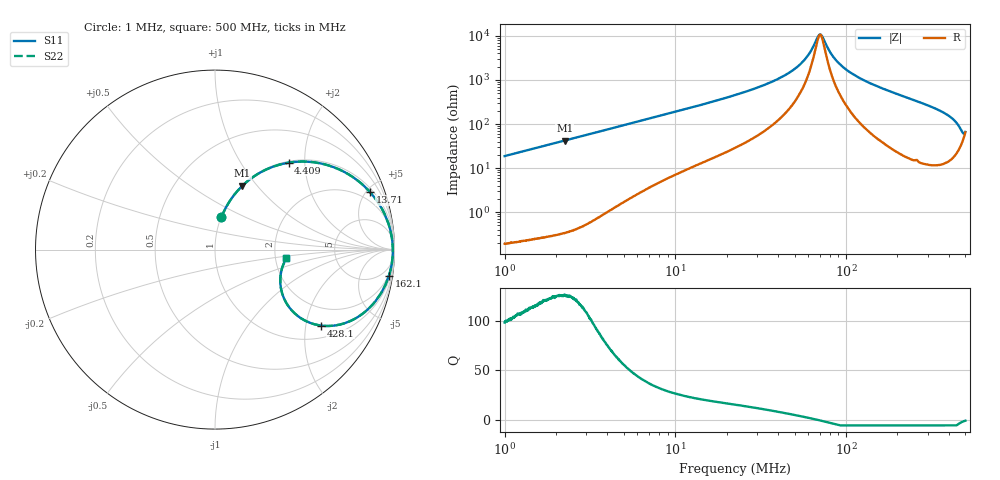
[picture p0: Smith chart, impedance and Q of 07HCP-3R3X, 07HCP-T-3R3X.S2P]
!s-Parameter Generated by FASTRON Sdn. Bhd.
!FASTRON P/N : 07HCP-3R3X, 07HCP/T-3R3X
!Keysight Technologies,E4991B,MY54100416,A.01.15
!Date: Fri Feb 20 12:59:01 2026
!Version  : Rev00 Fri Feb 20 12:59:01 2026
!Data & Calibration Information:
!PortZ  Port1:50+j0  Port2:50+j0
!When reading, reference impedance value at option line is always used.
! Remarks : This data is being provided solely for informational purposes.
!Freq	S11	S21	S12	S22
# Hz S dB R 50
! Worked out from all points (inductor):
!   1601 points, 1 MHz to 500 MHz, reference 50 ohm
!   read as one part in series: L = 2.98 uH near 1.032 MHz
!   highest Q = 125 at 2.252 MHz (marker M1), where L = 2.98 uH
!   self-resonance near 70.48 MHz
!   S11 on the Smith chart (normalised r, x): 1 MHz: 1.00, +0.37; 4.409 MHz: 1.03, +1.66; 13.71 MHz: 1.24, +5.26; 162.1 MHz: 2, -13; 428.1 MHz: 1.36, -2.45; 500 MHz: 2.30, -0.27
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1000000  -14.71 78.8  -0.17 -10.6  -0.17 -10.6  -14.71 78.8
2251920  -8.23 66.7  -0.74 -22.8  -0.74 -22.8  -8.23 66.7
2820919  -6.63 61.7  -1.10 -27.8  -1.10 -27.8  -6.63 61.7
4409396  -3.95 49.8  -2.34 -39.4  -2.34 -39.4  -3.95 49.8
7957584  -1.71 33.0  -5.27 -55.2  -5.27 -55.2  -1.71 33.0
1.370696e7  -0.72 20.4  -9.13 -66.9  -9.13 -66.9  -0.72 20.4
2.236068e7  -0.32 12.2  -13.46 -74.2  -13.46 -74.2  -0.32 12.2
4.481592e7  -0.11 4.2  -22.70 -77.8  -22.70 -77.8  -0.11 4.2
5.484648e7  -0.09 2.3  -27.81 -74.0  -27.81 -74.0  -0.09 2.3
6.307767e7  -0.08 1.0  -34.09 -60.7  -34.09 -60.7  -0.08 1.0
6.843836e7  -0.08 0.3  -39.73 -26.7  -39.73 -26.7  -0.08 0.3
7.11489e7  -0.08 -0.1  -40.65 9.2  -40.65 9.2  -0.08 -0.1
8.310792e7  -0.08 -1.5  -31.20 69.6  -31.20 69.6  -0.08 -1.5
9.520996e7  -0.09 -2.8  -26.19 76.8  -26.19 76.8  -0.09 -2.8
1.18344e8  -0.11 -4.9  -21.25 79.3  -21.25 79.3  -0.11 -4.9
1.620995e8  -0.18 -8.6  -16.46 77.9  -16.46 77.9  -0.18 -8.6
1.77937e8  -0.21 -9.9  -15.27 77.0  -15.27 77.0  -0.21 -9.9
3.186359e8  -0.82 -22.0  -8.53 65.3  -8.53 65.3  -0.82 -22.0
3.780214e8  -1.47 -28.5  -6.40 57.3  -6.40 57.3  -1.47 -28.5
4.280512e8  -2.75 -35.6  -4.62 46.1  -4.62 46.1  -2.75 -35.6
4.608356e8  -4.88 -38.7  -3.62 32.7  -3.62 32.7  -4.88 -38.7
5e8  -7.95 -7.1  -4.37 4.7  -4.37 4.7  -7.95 -7.1
